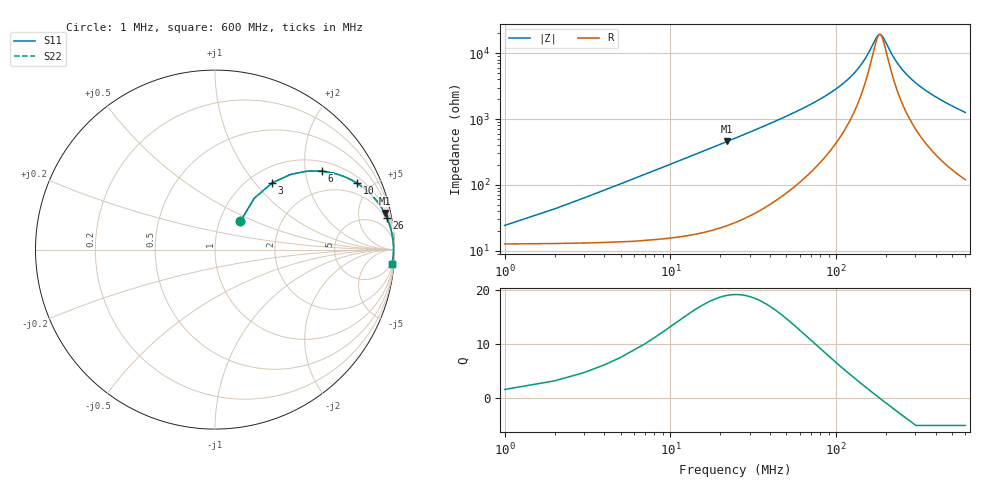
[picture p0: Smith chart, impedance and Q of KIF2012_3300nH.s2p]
!version-2
!date-12.2020
!Series
# MHz S RI R 50
!Freq ReS11 ImS11 ReS21 ImS21 ReS12 ImS12 ReS22 ImS22
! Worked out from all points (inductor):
!   600 points, 1 MHz to 600 MHz, reference 50 ohm
!   read as one part in series: L = 3.27 uH near 4 MHz
!   highest Q = 18.9 at 22 MHz (marker M1), where L = 3.3 uH
!   self-resonance near 182 MHz
!   S11 on the Smith chart (normalised r, x): 1 MHz: 1.25, +0.41; 3 MHz: 1.26, +1.24; 6 MHz: 1.28, +2.47; 10 MHz: 1.31, +4.11; 26 MHz: 2, +11; 600 MHz: 3, -25
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1  0.1414 0.1572  0.8586 -0.1572  0.8586 -0.1572  0.1414 0.1572
3  0.3189 0.3719  0.6811 -0.3719  0.6811 -0.3719  0.3189 0.3719
6  0.5956 0.4376  0.4044 -0.4376  0.4044 -0.4376  0.5956 0.4376
8  0.714 0.4093  0.286 -0.4093  0.286 -0.4093  0.714 0.4093
10  0.7917 0.3699  0.2083 -0.3699  0.2083 -0.3699  0.7917 0.3699
15  0.8918 0.2824  0.1082 -0.2824  0.1082 -0.2824  0.8918 0.2824
22  0.9444 0.2042  0.0556 -0.2042  0.0556 -0.2042  0.9444 0.2042
26  0.9586 0.1747  0.0414 -0.1747  0.0414 -0.1747  0.9586 0.1747
37  0.9774 0.1229  0.0226 -0.1229  0.0226 -0.1229  0.9774 0.1229
52  0.9867 0.0847  0.0133 -0.0847  0.0133 -0.0847  0.9867 0.0847
101  0.9937 0.0333  0.00633 -0.0333  0.00633 -0.0333  0.9937 0.0333
139  0.9946 0.0147  0.00536 -0.0147  0.00536 -0.0147  0.9946 0.0147
178  0.9948 0.00145  0.00517 -0.00145  0.00517 -0.00145  0.9948 0.00145
187  0.9948 -0.00116  0.00519 0.00116  0.00519 0.00116  0.9948 -0.00116
201  0.9948 -0.00498  0.00524 0.00498  0.00524 0.00498  0.9948 -0.00498
221  0.9946 -0.01  0.00537 0.01  0.00537 0.01  0.9946 -0.01
242  0.9944 -0.015  0.00555 0.015  0.00555 0.015  0.9944 -0.015
268  0.9942 -0.0207  0.00585 0.0207  0.00585 0.0207  0.9942 -0.0207
301  0.9937 -0.0274  0.00631 0.0274  0.00631 0.0274  0.9937 -0.0274
401  0.9918 -0.0457  0.00817 0.0457  0.00817 0.0457  0.9918 -0.0457
501  0.9893 -0.0622  0.0107 0.0622  0.0107 0.0622  0.9893 -0.0622
600  0.9863 -0.0776  0.0137 0.0776  0.0137 0.0776  0.9863 -0.0776
